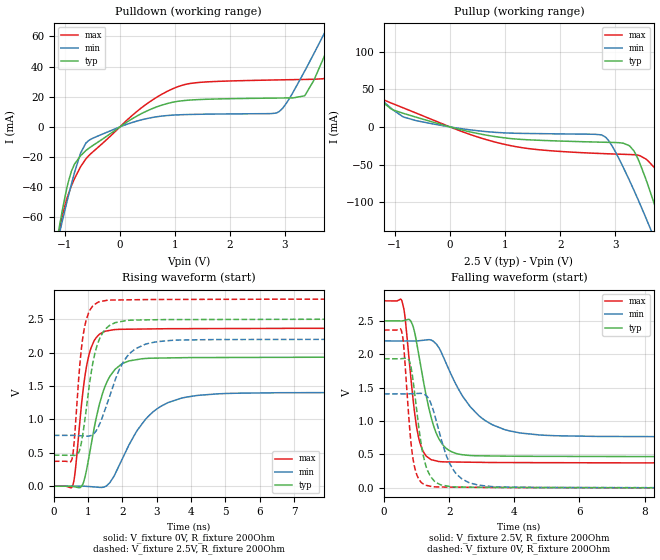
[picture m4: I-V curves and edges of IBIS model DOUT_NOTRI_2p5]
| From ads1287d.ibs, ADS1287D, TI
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|   Model
[Model]   DOUT_NOTRI_2p5
Model_type   Output
Polarity   Non-Inverting
Vmeas = 1.25
Vref = 0
Cref = 1pF
Rref = 100000
|   typ   min   max
C_comp   3.353pF   2.933pF   3.722pF
[Voltage Range]   2.5   2.2   2.8
[Temperature Range]   27   125   -40
[Pullup Reference]   2.5   2.2   2.8
[Pulldown Reference]   0   -0   0
[Power Clamp Reference]   2.5   2.2   2.8
[GND Clamp Reference]   0   0   0
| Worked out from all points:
|   slope of the pulldown table from 0 to 0.375 V, typ, clamps not added: 44.1 ohm
|   slope of the pullup table from 0 to 0.375 V, typ, clamps not added: 55.4 ohm
|   falling waveform, V_fixture 2.5V, R_fixture 200Ohm: 20-80 % time 531ps typ, 1.13ns min, 325ps max; typ from 2.5 V to 0.466 V
|   rising waveform, V_fixture 0V, R_fixture 200Ohm: 20-80 % time 530ps typ, 1.05ns min, 319ps max; typ from 0 V to 1.93 V
|   rising waveform, V_fixture 2.5V, R_fixture 200Ohm: 20-80 % time 381ps typ, 668ps min, 251ps max; typ from 0.466 V to 2.5 V
|   falling waveform, V_fixture 0V, R_fixture 200Ohm: 20-80 % time 347ps typ, 579ps min, 238ps max; typ from 1.93 V to 0 V
[Pulldown]
|   Voltage   I(typ)   I(min)   I(max)
-2.5V     -397.3mA   -325.7mA   -469.5mA
-1.09V    -64.11mA   -69.33mA   -67.16mA
-880mV    -29.29mA   -37.82mA   -38.97mA
-617.5mV  -15.63mA   -10.67mA   -21.14mA
327.5mV   7.586mA    4.071mA    10.8mA
882.5mV   15.71mA    7.63mA     23.98mA
1.377V    18.03mA    8.346mA    29.28mA
2.848V    19.13mA    9.306mA    31.15mA
3.357V    20.62mA    37.02mA    31.47mA
3.822V    56.43mA    69.79mA    36.28mA
4.152V    86.36mA    93.6mA     70.58mA
5V        165.1mA    155.5mA    169.7mA
[Pullup]
|   Voltage   I(typ)   I(min)   I(max)
-2.5V     148.5mA    125.8mA    179.2mA
-1.285V   38.53mA    38.87mA    41.44mA
-1.03V    22.46mA    22.33mA    30.63mA
-617.5mV  12.99mA    8.397mA    18.45mA
957.5mV   -14.25mA   -7.802mA   -22.64mA
2.757V    -20.29mA   -10.81mA   -35.41mA
2.953V    -20.63mA   -26.45mA   -35.94mA
3.26V     -25.1mA    -71.32mA   -36.68mA
3.59V     -76.34mA   -126.7mA   -44.62mA
3.853V    -134.4mA   -173.6mA   -75.44mA
4.122V    -197.4mA   -223.3mA   -146.3mA
5V        -411.2mA   -391.4mA   -401.8mA
[Ramp]
R_load = 200
|   typ   min   max
dV/dt_r   1.15988/5.29868e-10   0.844449/1.04274e-09   1.41824/3.18483e-10
dV/dt_f   1.22037/5.30711e-10   0.863306/1.12691e-09   1.45603/3.24225e-10
[Falling Waveform]
V_fixture = 2.5V
V_fixture_min = 2.2V
V_fixture_max = 2.8V
R_fixture = 200Ohm
C_fixture = 0F
|   Time   V(typ)   V(min)   V(max)
0s        2.5V       2.2V       2.8V
555.2ps   2.499V     2.2V       2.792V
645.7ps   2.51V      2.2V       2.555V
869.4ps   2.449V     2.2V       1.431V
1.011ns   2.148V     2.2V       881.6mV
1.159ns   1.738V     2.208V     592.8mV
1.676ns   743.7mV    2.105V     395mV
2.911ns   479.9mV    1.082V     382.2mV
4.788ns   472.1mV    791.6mV    377.5mV
50ns      466.1mV    761.2mV    373.3mV
[Rising Waveform]
V_fixture = 0V
V_fixture_min = 0V
V_fixture_max = 0V
R_fixture = 200Ohm
C_fixture = 0F
|   Time   V(typ)   V(min)   V(max)
0s        -643.4nV   -456.2nV   -98.41nV
566.2ps   -5.178mV   344.5uV    36.42mV
848.8ps   35.81mV    516.7uV    1.418V
987ps     334.7mV    -2.735mV   1.883V
1.159ns   825.1mV    -9.595mV   2.162V
1.425ns   1.398V     -15.67mV   2.302V
1.748ns   1.724V     145.4mV    2.343V
2.911ns   1.917V     1.121V     2.355V
4.788ns   1.926V     1.383V     2.36V
50ns      1.933V     1.407V     2.364V
[Rising Waveform]
V_fixture = 2.5V
V_fixture_min = 2.2V
V_fixture_max = 2.8V
R_fixture = 200Ohm
C_fixture = 0F
|   Time   V(typ)   V(min)   V(max)
0s        466.1mV    761.2mV    373.3mV
523.8ps   461.9mV    761.3mV    396.7mV
743.5ps   528.4mV    756.7mV    1.732V
853.5ps   809.7mV    752.9mV    2.256V
1.011ns   1.422V     749.4mV    2.592V
1.238ns   2.07V      834.1mV    2.737V
1.551ns   2.374V     1.234V     2.783V
2.232ns   2.485V     1.998V     2.79V
3.569ns   2.494V     2.186V     2.795V
50ns      2.5V       2.2V       2.8V
[Falling Waveform]
|Gnd
V_fixture = 0V
V_fixture_min = 0V
V_fixture_max = 0V
R_fixture = 200Ohm
C_fixture = 0F
|   Time   V(typ)   V(min)   V(max)
0s        1.933V     1.407V     2.364V
535ps     1.934V     1.407V     2.354V
607.8ps   1.938V     1.407V     2.106V
786.6ps   1.89V      1.408V     901.6mV
1.011ns   1.135V     1.413V     190.8mV
1.216ns   461.3mV    1.406V     56.06mV
1.497ns   129.5mV    1.187V     16.84mV
2.188ns   13.3mV     228.6mV    10.82mV
3.445ns   6.483mV    15.37mV    4.977mV
50ns      -495.3nV   -421nV     -64.46nV
